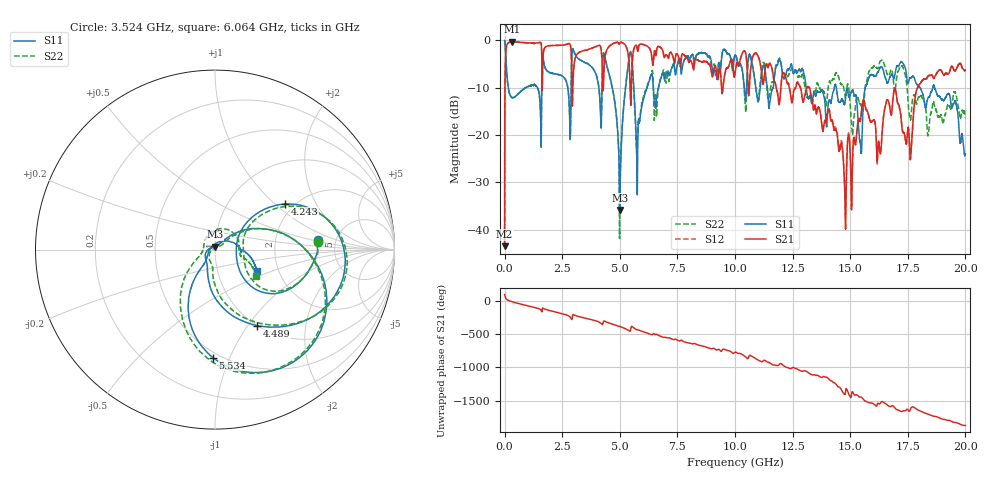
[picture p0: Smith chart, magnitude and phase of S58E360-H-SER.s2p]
!{S58E360}
!Johanson Technology Inc.
!www.johansontechnology.com
!Test Board Conditions:
!Substrate Type  RO4350B
!Substrate Thickness  60 mil
!Substrate Dk  3.66
!TL Type: GCPW
!TL Trace Width  115 mil
!TL Gap  52 mil
!Electrode orientation  Horizontal
!DUT TOPOLOGY	SERIES
!Mounting Pad LxW  55x428 mil
! Created Wed Apr 14 11:44:19 2021
# mhz S ma R 50
! 2 Port Network Data from SP1.SP block
! freq  magS11  angS11  magS21  angS21  magS12  angS12  magS22  angS22
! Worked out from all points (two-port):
!   20001 points, 300 kHz to 20 GHz, reference 50 ohm
!   highest |S21| = -0.28 dB at 328.3 MHz (marker M1); lowest = -43.5 dB at 300 kHz (marker M2)
!   |S21| within 3 dB of the highest: 42.38 MHz to 1.613 GHz (1.571 GHz wide, 190 % of centre); 1.671 GHz to 2.894 GHz (1.223 GHz wide, 53.6 % of centre)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
!   lowest |S11| = -35.8 dB at 4.993 GHz (marker M3), VSWR 1.03, Z = 49.8 + j1.6 ohm
!   |S11| at or under -10 dB: 13.09 GHz to 14.31 GHz (1.218 GHz wide, 8.89 % of centre); 14.4 GHz to 15.65 GHz (1.258 GHz wide, 8.37 % of centre); 18.67 GHz to end of sweep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
!   |S22| runs from -41.8 to 0.0 dB; largest |S21 - S12| = 0.0099
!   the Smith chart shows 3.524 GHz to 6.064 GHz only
!   S11 on the Smith chart (normalised r, x): 3.524 GHz: 3.63, +0.58; 4.243 GHz: 1.80, +1.16; 4.489 GHz: 1.00, -1.11; 5.534 GHz: 0.46, -0.87; 6.064 GHz: 1.55, -0.39
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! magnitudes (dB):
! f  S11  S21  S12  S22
! 300 kHz  -0.1  -43.5  -43.4  -0.1
! 108.3 MHz  -7.8  -0.8  -0.8  -7.8
! 328.3 MHz  -12.1  -0.3  -0.3  -12.1
! 2.79 GHz  -12.3  -0.7  -0.6  -12.3
! 3.334 GHz  -4.3  -2.3  -2.3  -4.3
! 3.524 GHz  -4.8  -2.1  -2.1  -4.8
! 4.243 GHz  -6.6  -5.5  -5.5  -6.2
! 4.489 GHz  -6.3  -1.6  -1.5  -6.2
! 4.993 GHz  -35.8  -0.6  -0.6  -38.8
! 5.534 GHz  -4.4  -5.4  -5.4  -4.6
! 5.76 GHz  -32.6  -1.8  -1.8  -21.7
! 6.064 GHz  -11.7  -0.9  -1.0  -11.3
! 6.667 GHz  -10.1  -1.3  -1.3  -10.5
! 10 GHz  -3.1  -7.0  -7.1  -3.2
! 13.33 GHz  -13.3  -12.1  -12.3  -12.8
! 14.77 GHz  -13.3  -32.5  -31.7  -11.5
! 15.44 GHz  -21.7  -17.0  -17.1  -13.5
! 16.25 GHz  -6.3  -21.5  -21.6  -5.3
! 16.67 GHz  -8.5  -12.9  -12.9  -7.3
! 17.61 GHz  -7.9  -25.1  -25.1  -16.7
! 18.07 GHz  -10.3  -8.9  -8.8  -11.7
! 20 GHz  -23.9  -6.2  -6.2  -16.4
